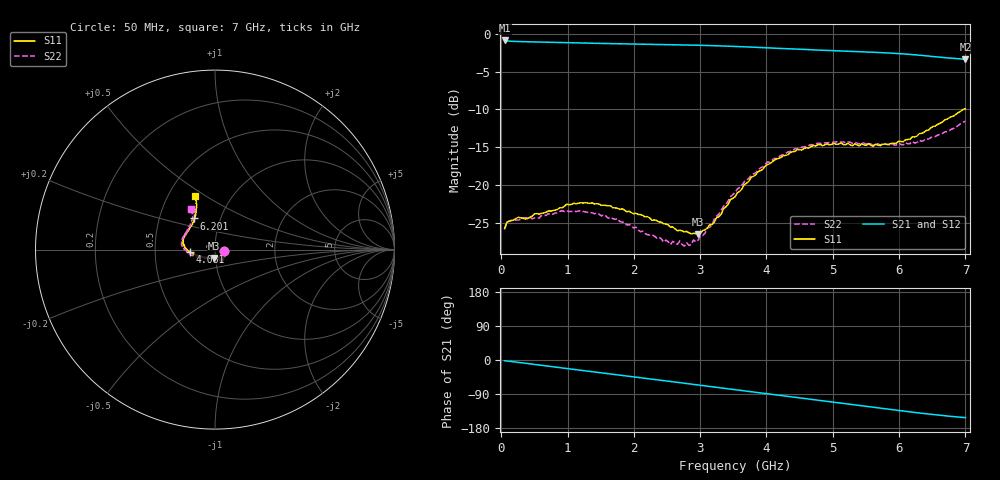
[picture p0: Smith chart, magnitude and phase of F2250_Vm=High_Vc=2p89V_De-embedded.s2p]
! Integrated Device Technology
! Corporate Headquarters
! 6024 Silver Creek Valley Road
! San Jose, CA 95138  USA
! Phone:  1-408-284-8200
! Toll Free:  1-800-223-1366
! Webpage:  http://www.idt.com/
! Timing and RF Division
! 515 Groton Road, Suite 102
! Westford, MA 01886-6024
! Device:  F2250
! Description: Voltage Variable RF Attenuator
! Frequency:  50.0 -  6000.00 MHz
! Package:  3x3 mm Thin QFN Plastic Package: 16 pin
! Ports:  2 RF, 3 DC
!  Pin  1  = GND
!  Pin  2  = NC
!  Pin  3  = RF1  = Port 1
!  Pin  4  = NC
!  Pin  5  = GND
!  Pin  6  = GND
!  Pin  7  = GND
!  Pin  8  = GND
!  Pin  9  = NC
!  Pin 10  = RF2  = Port 2
!  Pin 11  = NC
!  Pin 12  = GND
!  Pin 13  = GND
!  Pin 14  = VCNTRL
!  Pin 15  = VDD
!  Pin 16  = VMODE
! Vcntrl:  2.890 Volts
! Vmode:  +3.300 Volts
! Vdd:  +3.30  Volts
! Current:  1.313 mA
! Data:  The device was measured on a the F2250 evaluation board which has
!  individual transmission lines to the RF pins.  Data was collected
!  using a calibrated network analyzer.  The evaluation board was
!  de-embedded using a TRL calibration technique.
!  The reference plane is the edge of the package pin.
! Misc:  SN 10
!  Action Tracker AT0258
! Date Measured:  2014-11-26
! Date:  2015-10-15  MJV
! Note:
!  Integrated Device Technology supplies this data as a sample of measured
!  data at the package pin for this product.  Your particular data for this
!  product may vary.
!  Data was taken at 25 degrees C.
!  Integrated Device Technology reserves the right to change this data at anytime.
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# GHz S dB R 50
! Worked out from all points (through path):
!   201 points, 50 MHz to 7 GHz, reference 50 ohm
!   highest |S21| = -0.89 dB at 50 MHz (marker M1); lowest = -3.4 dB at 7 GHz (marker M2)
!   group delay of S21, straight-line fit = 61.2 ps
!   lowest |S11| = -26.5 dB at 2.969 GHz (marker M3), VSWR 1.10, Z = 49.1 - j4.62 ohm
!   |S11| at or under -10 dB: start of sweep to 6.967 GHz
!   |S22| runs from -28.0 to -11.5 dB; largest |S21 - S12| = 0.0019
!   S11 on the Smith chart (normalised r, x): 50 MHz: 1.11, -0.02; 4.081 GHz: 0.75, -0.02; 6.201 GHz: 0.75, +0.27; 7 GHz: 0.68, +0.45
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0.05  -25.69 -10.8  -0.89 -1.8  -0.89 -1.8  -25.84 -11.0
0.1195  -24.76 -10.1  -0.99 -3.2  -0.98 -3.2  -24.69 -8.8
0.57125  -23.84 -31.3  -1.10 -13.3  -1.10 -13.3  -24.33 -31.4
0.91875  -22.99 -50.1  -1.17 -21.0  -1.17 -21.1  -23.35 -51.0
1.2315  -22.36 -57.9  -1.24 -27.9  -1.24 -27.9  -23.47 -61.5
1.75275  -23.03 -64.8  -1.33 -39.1  -1.33 -39.1  -24.42 -67.8
2.37825  -24.86 -64.5  -1.42 -52.8  -1.42 -52.8  -26.86 -66.7
2.552  -25.52 -69.5  -1.44 -56.7  -1.44 -56.7  -27.84 -73.0
2.691  -25.93 -77.5  -1.47 -59.8  -1.47 -59.8  -27.37 -80.8
2.7605  -26.16 -79.8  -1.48 -61.3  -1.48 -61.3  -28.05 -85.2
2.969  -26.49 -97.8  -1.52 -66.0  -1.52 -66.0  -27.27 -104.8
3.1775  -25.21 -120.9  -1.57 -70.7  -1.57 -70.7  -25.24 -126.7
3.525  -21.54 -152.8  -1.68 -78.5  -1.68 -78.6  -20.97 -148.7
3.76825  -18.96 -164.8  -1.77 -84.0  -1.77 -84.1  -18.70 -159.6
4.081  -16.95 -175.7  -1.90 -91.0  -1.90 -91.0  -16.72 -171.4
4.4285  -15.54 176.0  -2.03 -98.6  -2.04 -98.7  -15.19 178.7
4.7065  -14.76 169.1  -2.13 -104.8  -2.13 -104.8  -14.68 173.0
5.054  -14.60 160.9  -2.26 -112.5  -2.25 -112.5  -14.27 166.0
5.85325  -14.57 135.1  -2.56 -130.0  -2.56 -130.1  -14.67 147.3
6.20075  -13.62 123.6  -2.77 -137.7  -2.77 -137.8  -14.24 138.2
6.54825  -12.18 115.6  -3.04 -144.7  -3.04 -144.9  -13.58 126.9
7  -9.91 110.7  -3.36 -152.1  -3.37 -152.2  -11.54 120.7
